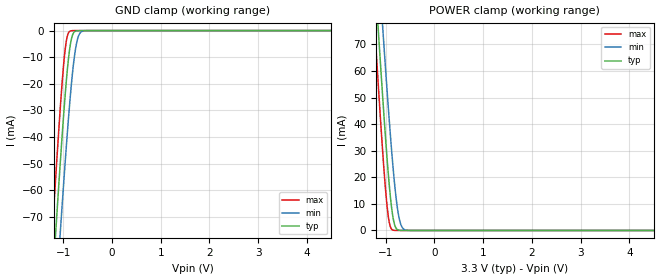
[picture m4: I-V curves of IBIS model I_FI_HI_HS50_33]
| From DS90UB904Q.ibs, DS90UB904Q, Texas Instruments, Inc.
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|   I_FI_HI_HS50_33   Input model
[Model]   I_FI_HI_HS50_33
Model_type   Input
Vinl = 0.8V
Vinh = 2.0V
|   typ   min   max
|   (nom)   (weak)   (strong)
C_comp   0.6368pF   0.6368pF   0.6368pF
[Voltage Range]   3.300V   3.000V   3.600V
[Temperature Range]   25.0   105.0   -40.0
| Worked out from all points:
|   GND clamp passes 1 mA (typ) near -0.79 V on its own axis
|   POWER clamp passes 1 mA (typ) near -0.79 V on its own axis
[GND Clamp]
|   Voltage   I(typ)   I(min)   I(max)
-3.3V     -738.9mA   -744.2mA   -736.5mA
-1.231V   -97.79mA   -123.3mA   -77.52mA
-1.221V   -94.89mA   -120.4mA   -74.56mA
-1.171V   -80.54mA   -106.4mA   -59.92mA
-1.142V   -72.04mA   -98.1mA    -51.31mA
-1.063V   -50mA      -76.27mA   -29.42mA
-953.7mV  -22.55mA   -47.66mA   -6.049mA
-914.1mV  -14.3mA    -37.94mA   -1.919mA
-854.7mV  -5.238mA   -24.54mA   -154.3uA
-735.9mV  -128.9uA   -5.576mA   -5.191uA
-597.3mV  -3.652uA   -175.8uA   -4.75uA
6.59V     0A         0A         0A
[POWER Clamp]
|   Voltage   I(typ)   I(min)   I(max)
-3.3V     739mA      744.2mA    736.5mA
-1.231V   97.81mA    123.3mA    77.54mA
-1.221V   94.91mA    120.5mA    74.58mA
-1.171V   80.56mA    106.5mA    59.94mA
-1.142V   72.06mA    98.13mA    51.33mA
-1.063V   50.02mA    76.29mA    29.44mA
-953.7mV  22.57mA    47.69mA    6.067mA
-914.1mV  14.32mA    37.97mA    1.933mA
-854.7mV  5.262mA    24.57mA    156.8uA
-735.9mV  134.2uA    5.608mA    2.976uA
-597.3mV  2.162uA    187.4uA    2.024uA
6.59V     0A         0A         0A
